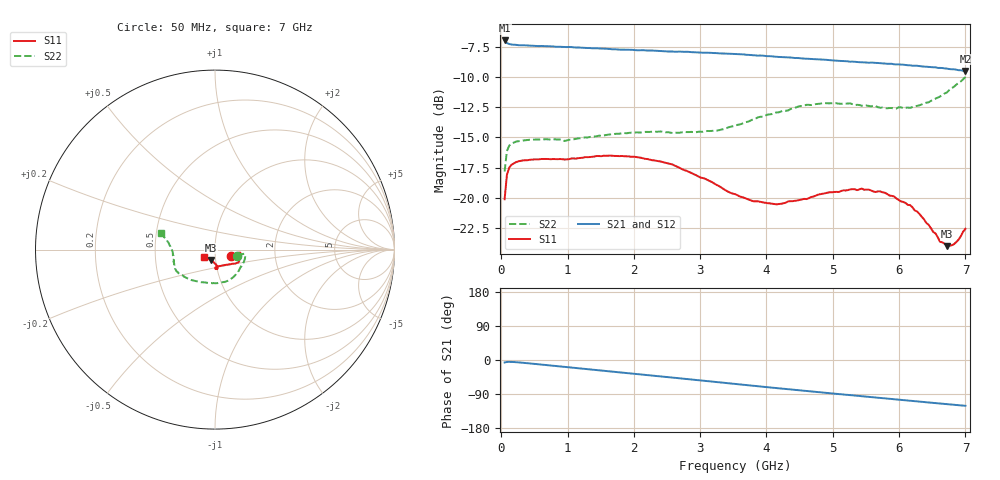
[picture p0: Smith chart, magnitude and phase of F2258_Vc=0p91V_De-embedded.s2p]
! Integrated Device Technology
! Corporate Headquarters
! 6024 Silver Creek Valley Road
! San Jose, CA 95138  USA
! Phone:  1-408-284-8200
! Toll Free:  1-800-223-1366
! Webpage:  http://www.idt.com/
! Timing and RF Division
! 515 Groton Road, Suite 102
! Westford, MA 01886-6024
! Device:  F2258
! Description: Voltage Variable RF Attenuator
! Frequency:  50.0 -  6000.00 MHz
! Package:  3x3 mm Thin QFN Plastic Package: 16 pin
! Ports:  2 RF, 2 DC
!  Pin  1  = NC
!  Pin  2  = NC
!  Pin  3  = RF2  = Port 2
!  Pin  4  = GND
!  Pin  5  = Vdd
!  Pin  6  = NC
!  Pin  7  = VCTRL
!  Pin  8  = NC
!  Pin  9  = GND
!  Pin 10  = RF1  = Port 1
!  Pin 11  = NC
!  Pin 12  = NC
!  Pin 13  = NC
!  Pin 14  = NC
!  Pin 15  = NC
!  Pin 16  = NC
! Vcntrl:  0.910 Volts
! Vdd:  +3.300 Volts
! Current:  1.147 mA
! Data:  The device was measured on a the F2258 evaluation board which has
!  individual transmission lines to the RF pins.  Data was collected
!  using a calibrated network analyzer.  The evaluation board was
!  de-embedded using a TRL calibration technique.
!  The reference plane is the edge of the package pin.
! Misc:  SN 10
!  Action Tracker AT0285
! Date Measured:  2014-12-10
! Date:  2016-01-13  MJV
! Note:
!  Integrated Device Technology supplies this data as a sample of measured
!  data at the package pin for this product.  Your particular data for this
!  product may vary.
!  Data was taken at 25 degrees C.
!  Integrated Device Technology reserves the right to change this data at anytime.
!Freq_(GHz)  S11M_(dB)  S11P_(deg)  S21M_(dB)  S21P_(deg)  S12M_(dB)  S12P_(deg)  S22M_(dB)  S22P_(deg)
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# GHz S dB R 50
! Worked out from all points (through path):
!   201 points, 50 MHz to 7 GHz, reference 50 ohm
!   highest |S21| = -6.98 dB at 50 MHz (marker M1); lowest = -9.5 dB at 7 GHz (marker M2)
!   group delay of S21, straight-line fit = 47.6 ps
!   lowest |S11| = -24.0 dB at 6.722 GHz (marker M3), VSWR 1.13, Z = 47.3 - j5.53 ohm
!   |S11| at or under -10 dB: start of sweep to end of sweep
!   |S22| runs from -17.8 to -10.0 dB; largest |S21 - S12| = 0.0018
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0.05  -20.12 -22.9  -6.98 -6.6  -6.96 -6.6  -17.81 -15.5
0.08475  -18.10 -11.1  -7.19 -5.1  -7.19 -5.1  -16.13 -9.0
0.1195  -17.50 -7.9  -7.27 -4.9  -7.27 -4.9  -15.68 -8.2
0.22375  -17.04 -6.8  -7.34 -5.8  -7.34 -5.8  -15.35 -9.6
0.9535  -16.83 -18.6  -7.52 -18.2  -7.51 -18.2  -15.30 -33.2
1.2315  -16.68 -21.9  -7.58 -23.1  -7.58 -23.1  -15.03 -41.9
1.82225  -16.54 -27.5  -7.73 -33.3  -7.72 -33.3  -14.65 -58.1
2.37825  -16.98 -31.9  -7.84 -42.9  -7.87 -42.8  -14.52 -73.5
3.0385  -18.36 -41.7  -7.99 -54.4  -8.00 -54.4  -14.54 -95.8
3.525  -19.69 -55.8  -8.10 -63.1  -8.13 -63.1  -14.04 -115.2
3.803  -20.29 -67.0  -8.20 -68.1  -8.24 -68.1  -13.49 -125.7
4.1505  -20.54 -78.3  -8.33 -74.1  -8.34 -74.1  -12.93 -136.2
4.7065  -19.90 -88.4  -8.53 -83.6  -8.51 -83.6  -12.30 -149.0
5.2625  -19.30 -87.8  -8.73 -92.7  -8.71 -92.7  -12.18 -158.0
5.43625  -19.23 -85.6  -8.78 -95.5  -8.77 -95.5  -12.38 -160.9
5.85325  -19.80 -82.2  -8.91 -102.3  -8.91 -102.3  -12.57 -169.4
6.166  -20.60 -82.8  -9.04 -107.4  -9.04 -107.4  -12.56 -176.7
6.444  -22.22 -90.2  -9.16 -112.0  -9.18 -112.0  -12.10 176.1
6.61775  -23.64 -101.6  -9.25 -114.8  -9.25 -114.9  -11.62 171.4
6.722  -24.00 -112.6  -9.30 -116.6  -9.33 -116.5  -11.28 168.7
6.861  -23.67 -130.6  -9.39 -118.8  -9.41 -118.7  -10.65 166.0
7  -22.57 -147.8  -9.51 -120.9  -9.51 -120.9  -10.00 163.3
